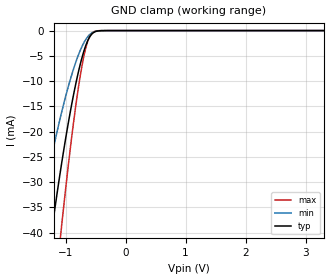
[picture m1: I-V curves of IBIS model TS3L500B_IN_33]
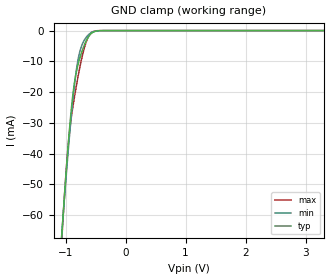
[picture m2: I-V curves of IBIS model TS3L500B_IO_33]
| TEXAS INSTRUMENTS INCORPORATED
| Standard Linear and Logic Group
| IBIS Model of TS3L500
| 16-Bit to 8-Bit SPDT Gigabit LAN Switch with LED Switch
| This file contains package information for the following:
|  QFN 56-pin (QFN) package as [Component] TS3L500B_QFN
| This device can be powered at the following Vccs:
|  3.3 volt Vcc
| This file provides unique models under the [Model Selector] for each Vcc.
| For operation at a specific Vcc, select the appropriate model after each
| [Model Selector] keyword.
[IBIS Ver]   3.2
[Comment char]  |_char
[File Name]   ts3l500.ibs
[File Rev]   1.1 | b_die
[Date]   July 21, 2005
[Source]   Data created from TI-SPICE simulations at TI-SLL.
[Notes]   The following is an IBIS list for the TS3L500B.
   Please contact sllibis@ti.com with questions and
   comments concerning SLL IBIS models.
   - FILE REV HISTORY
   - 1.1 Release IBIS file on 10/15/08
   - Power clamp data deleted was deleted as there is no
   power-clamp diode.
[Disclaimer] Property of Texas Instruments Incorporated.  Unauthorized
   reproduction and/or distribution is strictly prohibited.
   This product is protected under copyright law.
   Created  2005, (C) Copyright  2005, Texas Instruments
   Incorporated, All Rights Reserved
   UNLESS THERE IS A SIGNED, WRITTEN AGREEMENT TO THE
   CONTRARY, TEXAS INSTRUMENTS (TI) IS PROVIDING THE IBIS
   MODELS  AND WITHOUT ANY WARRANTY, EXPRESSED OR
   IMPLIED.  TI assumes no liability for:
   1) the accuracy of the IBIS models provided to your
   company;
   2) the proper functioning of these IBIS Models in your
   design or for any resulting applications; or
   3) infringement of patents, copyrights or intellectual
   property rights resulting from your use of these IBIS
   models.
   TI provides IBIS Models as a service to our customers.
   You and your company shall not distribute, sell or give
   these models to anyone else without prior written
   permission from TI.
   TI reserves the right to make changes to our products or
   to discontinue any semiconductor product or service
   without notice, and advises our customers to obtain the
   latest version of relevant information to verify, before
   placing orders, that the information being relied on is
   current.
   Please be aware that your receipt and use of the IBIS
   information provided shall serve as acceptance of these
   terms and conditions.  If you do not accept these terms,
   you should return or destroy the IBIS models and any
   other accompanying information immediately.
| Component TS3L500B_QFN 56-pin QFN
[Component]   TS3L500B_QFN
[Manufacturer]   Texas Instruments, Inc.
[Package]
|   typ   min   max
R_pkg   6.800e-02   0.000e+00   9.400e-02
L_pkg   2.215e-09   3.400e-11   3.050e-09
C_pkg   3.710e-13   1.950e-13   4.500e-13
[Pin]   signal_name   model_name   R_pin   L_pin   C_pin
1   GND   GND   8.700e-02   2.814e-09   4.360e-13
2   0A   TS3L500B_IO   8.900e-02   2.874e-09   4.190e-13
3   1A   TS3L500B_IO   8.300e-02   2.685e-09   4.020e-13
4   VCC   POWER   7.400e-02   2.399e-09   3.730e-13
5   NC   NC   0.000e+00   3.400e-11   1.950e-13
6   GND   GND   5.900e-02   1.937e-09   3.460e-13
7   2A   TS3L500B_IO   5.900e-02   1.915e-09   3.480e-13
8   3A   TS3L500B_IO   5.600e-02   1.825e-09   3.380e-13
9   GND   GND   4.900e-02   1.608e-09   3.230e-13
10   VCC   POWER   4.700e-02   1.549e-09   3.190e-13
11   4A   TS3L500B_IO   5.100e-02   1.652e-09   3.260e-13
12   5A   TS3L500B_IO   5.100e-02   1.667e-09   3.250e-13
13   GND   GND   4.900e-02   1.600e-09   3.200e-13
14   6A   TS3L500B_IO   5.500e-02   1.787e-09   3.350e-13
15   7A   TS3L500B_IO   5.800e-02   1.893e-09   3.460e-13
16   GND   GND   5.800e-02   1.889e-09   3.490e-13
17   SEL   TS3L500B_IN   6.300e-02   2.055e-09   3.630e-13
18   VCC   POWER   6.900e-02   2.240e-09   3.760e-13
19   0LED   TS3L500B_IO   7.400e-02   2.416e-09   3.870e-13
20   1LED   TS3L500B_IO   8.100e-02   2.614e-09   4.270e-13
21   GND   GND   8.200e-02   2.661e-09   4.310e-13
22   0LED1   TS3L500B_IO   7.800e-02   2.537e-09   4.000e-13
23   1LED1   TS3L500B_IO   7.500e-02   2.448e-09   3.940e-13
24   GND   GND   7.400e-02   2.392e-09   3.890e-13
25   0LED2   TS3L500B_IO   7.400e-02   2.387e-09   3.890e-13
26   1LED2   TS3L500B_IO   7.500e-02   2.418e-09   3.920e-13
27   VCC   POWER   7.700e-02   2.493e-09   3.940e-13
28   GND   GND   9.200e-02   2.981e-09   4.500e-13
29   7B2   TS3L500B_IO   9.400e-02   3.050e-09   4.500e-13
30   6B2   TS3L500B_IO   8.900e-02   2.883e-09   4.110e-13
31   7B1   TS3L500B_IO   8.300e-02   2.702e-09   4.000e-13
32   6B1   TS3L500B_IO   7.700e-02   2.505e-09   3.860e-13
33   GND   GND   7.100e-02   2.306e-09   3.710e-13
34   5B2   TS3L500B_IO   6.500e-02   2.120e-09   3.570e-13
35   4B2   TS3L500B_IO   5.900e-02   1.927e-09   3.430e-13
36   5B1   TS3L500B_IO   5.400e-02   1.759e-09   3.300e-13
37   4B1   TS3L500B_IO   5.000e-02   1.632e-09   3.210e-13
38   VCC   POWER   4.700e-02   1.550e-09   3.150e-13
39   GND   GND   4.700e-02   1.535e-09   3.140e-13
40   3B2   TS3L500B_IO   4.900e-02   1.589e-09   3.170e-13
41   2B2   TS3L500B_IO   5.200e-02   1.695e-09   3.250e-13
42   3B1   TS3L500B_IO   5.700e-02   1.845e-09   3.370e-13
43   2B1   TS3L500B_IO   6.200e-02   2.025e-09   3.500e-13
44   GND   GND   6.800e-02   2.203e-09   3.630e-13
45   1B2   TS3L500B_IO   7.400e-02   2.396e-09   3.770e-13
46   0B2   TS3L500B_IO   8.000e-02   2.588e-09   3.910e-13
47   1B1   TS3L500B_IO   8.500e-02   2.765e-09   4.030e-13
48   0B1   TS3L500B_IO   9.000e-02   2.930e-09   4.380e-13
49   GND   GND   8.800e-02   2.852e-09   4.380e-13
50   VCC   POWER   7.700e-02   2.502e-09   3.920e-13
51   2LED2   TS3L500B_IO   7.500e-02   2.428e-09   3.890e-13
52   2LED1   TS3L500B_IO   7.400e-02   2.388e-09   3.870e-13
53   GND   GND   7.400e-02   2.386e-09   3.860e-13
54   2LED   TS3L500B_IO   7.500e-02   2.425e-09   3.890e-13
55   GND   GND   7.700e-02   2.500e-09   3.930e-13
56   VCC   POWER   8.600e-02   2.780e-09   4.360e-13
[Series Switch Groups]
| Function Group States
On  1 /   | 0A-7A->0B1-7B1 SEL LOW
   | 0LED-1LED->0LED1-1LED1 SEL HIGH
On  2 /   | 0A-7A->0B2-7B2 SEL HIGH
   | 0LED-1LED->0LED2-1LED2 SEL HIGH
[Series Pin Mapping]   pin_2   model_name   function_table_group
2   48   TS3L500B_IO_33_S   1
3   47   TS3L500B_IO_33_S   1
7   43   TS3L500B_IO_33_S   1
8   42   TS3L500B_IO_33_S   1
11   37   TS3L500B_IO_33_S   1
12   36   TS3L500B_IO_33_S   1
14   32   TS3L500B_IO_33_S   1
15   31   TS3L500B_IO_33_S   1
19   22   TS3L500B_IO_33_S   1
20   23   TS3L500B_IO_33_S   1
2   46   TS3L500B_IO_33_S   2
3   45   TS3L500B_IO_33_S   2
7   41   TS3L500B_IO_33_S   2
8   40   TS3L500B_IO_33_S   2
11   35   TS3L500B_IO_33_S   2
12   34   TS3L500B_IO_33_S   2
14   30   TS3L500B_IO_33_S   2
15   29   TS3L500B_IO_33_S   2
19   25   TS3L500B_IO_33_S   2
20   26   TS3L500B_IO_33_S   2
| Model TS3L500B_IN
[Model Selector]   TS3L500B_IN
TS3L500B_IN_33   3.3 volt Vcc
| Model TS3L500B_IO
[Model Selector]   TS3L500B_IO
TS3L500B_IO_33   3.3 volt Vcc
[Model]   TS3L500B_IO_33_S
Model_type  Series_switch
Vref =   0
Rref =   200
Cref =   10p
Vmeas =   1.25
| variable   typ   min   max
C_comp   0   0   0
[Temperature Range]   40   100   -40
| Ambient temperature   25   85   -40
[Voltage range]   3.3   3   3.6
[On]
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[Off]
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| Models and submodels in the file (3): TS3L500B_IN_33 (Input), TS3L500B_IO_33_S (Series_switch), TS3L500B_IO_33 (Terminator)
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[Model]   TS3L500B_IN_33
Model_type  Input
Vinl=0.8
Vinh=2.0
| variable   typ   min   max
C_comp   1.72pF   1.44pF   1.89pF
[Temperature Range]   40   100   -40
| Ambient temperature   25   85   -40
[Voltage range]   3.3   3   3.6
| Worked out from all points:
|   GND clamp passes 1 mA (typ) near -0.58 V on its own axis
[GND Clamp]
| TS3L500B_IN_33
|   Voltage   I(typ)   I(min)   I(max)
-3.3V     -274.7mA   -196.9mA   -361.3mA
-1.48V    -62.72mA   -40.36mA   -90.68mA
-1.44V    -58.83mA   -37.71mA   -85.28mA
-1.235V   -40.09mA   -25.15mA   -58.77mA
-1.08V    -27.44mA   -16.9mA    -40.34mA
-1.065V   -26.29mA   -16.16mA   -38.64mA
-885mV    -13.83mA   -8.297mA   -19.91mA
-750mV    -6.446mA   -3.791mA   -8.618mA
-640mV    -2.264mA   -1.364mA   -2.471mA
-590mV    -1.113mA   -709.9uA   -1.005mA
-525mV    -329.9uA   -241.8uA   -213.8uA
3.3V      155.4pA    484.7pA    28.88pA
[Model]   TS3L500B_IO_33
Model_type  Terminator
| variable   typ   min   max
C_comp   2.55pF   2.30pF   2.82pF
| C_tri-state   2.55pF   2.30pF   2.82pF
[Temperature Range]   40   100   -40
| Ambient temperature   25   85   -40
[Voltage range]   3.3   3   3.6
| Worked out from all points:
|   GND clamp passes 1 mA (typ) near -0.57 V on its own axis
[GND Clamp]
| TS3L500B_IO_33
|   Voltage   I(typ)   I(min)   I(max)
-3.3V     -901.9mA   -814.6mA   -996.2mA
-1.07V    -68.79mA   -68.13mA   -70.43mA
-1.055V   -64.36mA   -64.15mA   -65.45mA
-990mV    -46.07mA   -47.52mA   -45.71mA
-945mV    -34.64mA   -36.76mA   -35.08mA
-870mV    -19.62mA   -20.99mA   -23.82mA
-805mV    -12.13mA   -10.97mA   -16.38mA
-740mV    -7.57mA    -5.41mA    -9.905mA
-665mV    -3.743mA   -2.427mA   -4.204mA
-600mV    -1.553mA   -1.056mA   -1.35mA
-540mV    -512uA     -393.9uA   -314.9uA
3.3V      225.3pA    927.9pA    33.95pA
